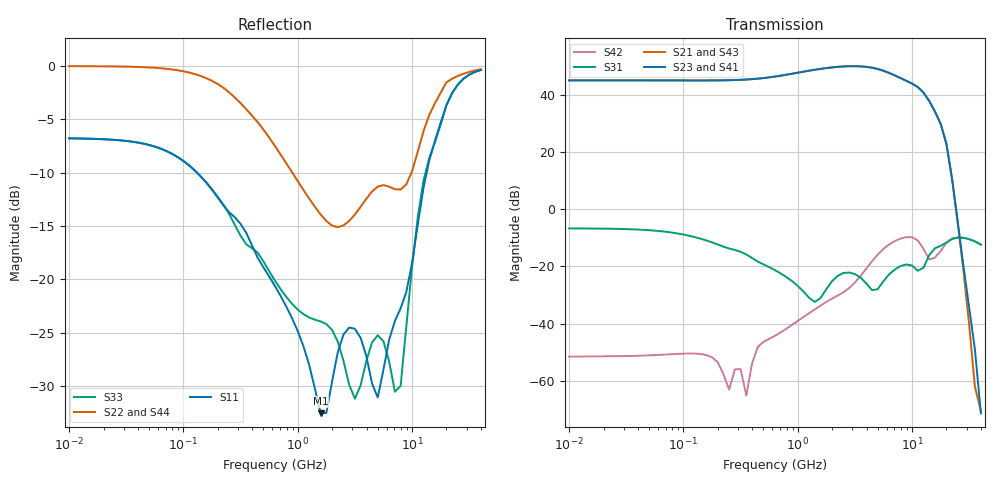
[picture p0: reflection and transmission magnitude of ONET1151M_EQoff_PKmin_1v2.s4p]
! Touchstone Ver. 1.0
! Thu Sep  6 15:30:02 2012
! Number of ports is 4
# Hz	S	DB	R	50.000000
! SCATTERING PARAMETERS  :
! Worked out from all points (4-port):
!   73 points, 10 MHz to 40 GHz, reference 50 ohm
!   strongest paths, dB at 10 MHz, 79.43 MHz, 631 MHz, 5.012 GHz, 40 GHz:
!     S23: 45.0, 45.0, 46.3, 48.9, -71.3
!     S21: 45.0, 45.0, 46.3, 48.9, -70.5
!     S43: 45.0, 45.0, 46.3, 48.8, -70.8
!     S41: 45.0, 45.0, 46.3, 48.8, -71.9
!     S31: -6.7, -8.2, -21.3, -27.9, -12.4
!     S42: -51.5, -50.6, -44.2, -15.8, -12.4
!   lowest |S11| = -32.5 dB at 1.585 GHz (marker M1), VSWR 1.05, Z = 51.2 - j2.05 ohm
!   |S11| at or under -10 dB: 131.2 MHz to 13.46 GHz (13.33 GHz wide, 196 % of centre)
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1e7  -6.80 -4.5  -110.51 177.0  -6.73 -4.3  -110.48 177.0
     44.97 -175.6  -0.04 7.1  44.97 4.4  -51.55 9.8
     -6.73 -4.3  -110.50 176.9  -6.80 -4.5  -110.50 177.0
     44.96 4.4  -51.49 9.8  44.96 -175.6  -0.04 7.1
1.584893e9  -32.55 -57.9  -40.79 67.0  -25.99 -53.9  -40.72 67.0
            48.99 127.8  -13.92 -84.5  48.99 -52.2  -37.45 39.0
            -31.01 2.4  -40.75 67.1  -23.94 -77.4  -40.73 67.0
            48.93 -52.6  -33.66 28.4  48.92 127.4  -13.95 -82.1
3.981072e9  -27.18 -112.5  -38.52 -10.1  -26.68 36.1  -38.46 -9.9
            49.69 7.8  -12.45 -113.9  49.68 -172.2  -20.19 -131.3
            -25.96 -89.6  -38.49 -9.7  -27.63 61.3  -38.45 -10.1
            49.58 -172.7  -20.73 -136.0  49.57 7.2  -12.75 -115.3
5.623413e9  -28.45 93.4  -37.96 -30.7  -34.23 -2.2  -37.91 -30.4
            48.33 -70.4  -11.18 -161.6  48.32 109.6  -13.25 157.0
            -25.16 128.8  -37.94 -30.3  -25.81 -7.9  -37.89 -30.7
            48.18 109.2  -13.87 156.6  48.16 -70.8  -11.55 -160.0
7.943282e9  -22.72 29.8  -38.46 -62.5  -22.54 89.8  -38.43 -62.0
            45.77 -172.3  -11.60 143.3  45.75 7.7  -10.08 90.8
            -19.88 70.5  -38.47 -61.8  -29.98 27.9  -38.38 -62.5
            45.63 7.4  -10.27 92.5  45.60 -172.5  -11.46 144.9
1.122018e10  -14.86 22.6  -40.35 -98.9  -19.22 55.0  -40.37 -97.7
             42.63 42.8  -8.05 79.0  42.62 -136.9  -11.04 28.0
             -21.50 46.9  -40.41 -97.3  -14.18 30.1  -40.29 -99.2
             42.51 -137.5  -10.91 27.6  42.48 42.7  -8.01 77.4
4e10  -0.40 -143.6  -68.64 141.6  -12.37 -52.7  -68.45 141.4
      -70.45 -150.2  -0.33 -143.9  -71.29 58.0  -12.41 -53.2
      -12.37 -52.7  -68.37 141.1  -0.40 -143.5  -68.63 141.8
      -71.90 60.6  -12.40 -53.3  -70.81 -149.4  -0.33 -143.9
